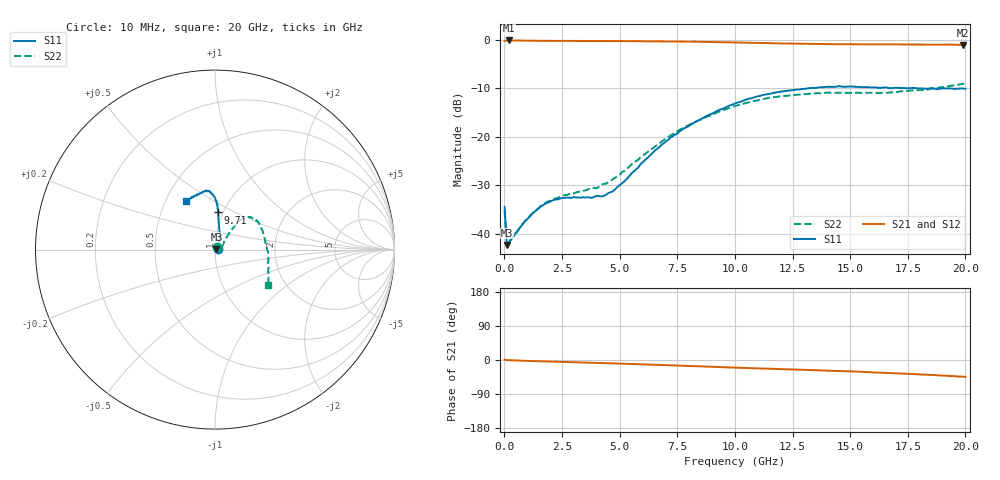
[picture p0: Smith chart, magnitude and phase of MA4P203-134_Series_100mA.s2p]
! AWR Design Environment (9226) Thu Aug 19 14:29:25 2021
! Document = '100mA'
! nPorts: 2, nXvals: 201
# GHz S DB R 50
!Freq DBS11 AngS11 DBS21 AngS21 DBS12 AngS12 DBS22 AngS22
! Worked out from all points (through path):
!   201 points, 10 MHz to 20 GHz, reference 50 ohm
!   highest |S21| = -0.12 dB at 210 MHz (marker M1); lowest = -1.0 dB at 19.91 GHz (marker M2)
!   group delay of S21, straight-line fit = 5.9 ps
!   lowest |S11| = -42.3 dB at 110 MHz (marker M3), VSWR 1.02, Z = 50.8 + j0.0684 ohm
!   |S11| at or under -10 dB: start of sweep to 13.16 GHz; 18.15 GHz to 18.44 GHz (288 MHz wide, 1.57 % of centre); 19.33 GHz to 19.78 GHz (451.9 MHz wide, 2.31 % of centre)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
!   |S22| runs from -42.5 to -9.0 dB; largest |S21 - S12| = 0.043
!   S11 on the Smith chart (normalised r, x): 10 MHz: 1.04, +0.01; 9.71 GHz: 0.95, +0.41; 20 GHz: 0.64, +0.38
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0.01  -34.47 18.0  -0.19 1.0  -0.17 0.7  -35.24 44.8
0.11  -42.28 5.0  -0.12 -0.3  -0.11 -0.3  -42.52 6.2
0.21  -41.66 7.8  -0.12 -0.5  -0.11 -0.5  -41.51 9.5
0.91  -37.32 2.4  -0.15 -2.1  -0.14 -2.0  -37.29 4.7
1.61  -34.25 -10.3  -0.19 -3.4  -0.18 -3.2  -34.11 -7.9
2.21  -32.90 -17.8  -0.21 -4.5  -0.20 -4.1  -32.69 -14.2
3.41  -32.42 -11.4  -0.23 -6.6  -0.22 -6.1  -31.10 -9.1
3.81  -32.52 -2.2  -0.24 -7.3  -0.22 -6.7  -30.62 -2.5
4.01  -32.12 3.0  -0.23 -7.7  -0.22 -7.1  -30.60 2.2
4.21  -32.29 12.5  -0.24 -8.0  -0.22 -7.5  -29.85 5.7
4.71  -31.21 29.3  -0.25 -8.9  -0.23 -8.3  -28.69 15.6
6.71  -22.14 71.2  -0.29 -13.0  -0.26 -12.2  -21.38 45.1
7.81  -18.18 79.2  -0.35 -15.4  -0.34 -14.4  -18.00 49.3
9.71  -13.64 85.4  -0.50 -19.4  -0.49 -18.2  -14.11 49.7
10.01  -13.11 85.4  -0.53 -20.2  -0.52 -18.8  -13.63 49.7
11.21  -11.36 88.1  -0.64 -22.7  -0.64 -21.0  -12.22 46.7
13.41  -9.91 94.6  -0.83 -26.6  -0.79 -25.0  -11.04 36.5
14.51  -9.53 98.2  -0.89 -29.1  -0.83 -27.0  -10.87 29.3
16.71  -9.96 108.9  -0.92 -34.5  -0.84 -32.1  -10.86 4.7
18.21  -10.02 117.1  -0.97 -38.3  -0.87 -36.8  -10.35 -14.3
19.91  -10.05 121.7  -1.04 -44.0  -0.97 -42.7  -9.04 -32.4
20  -10.06 120.5  -1.03 -44.6  -0.97 -43.0  -8.96 -33.3
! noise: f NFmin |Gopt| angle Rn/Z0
0.01  0  1  0  2e-20
2.21  0  1  0  2e-20
4.41  0  1  0  2e-20
6.61  0  1  0  2e-20
8.81  0  1  0  2e-20
11.11  0  1  0  2e-20
13.31  0  1  0  2e-20
15.51  0  1  0  2e-20
17.71  0  1  0  2e-20
20  0  1  0  2e-20
